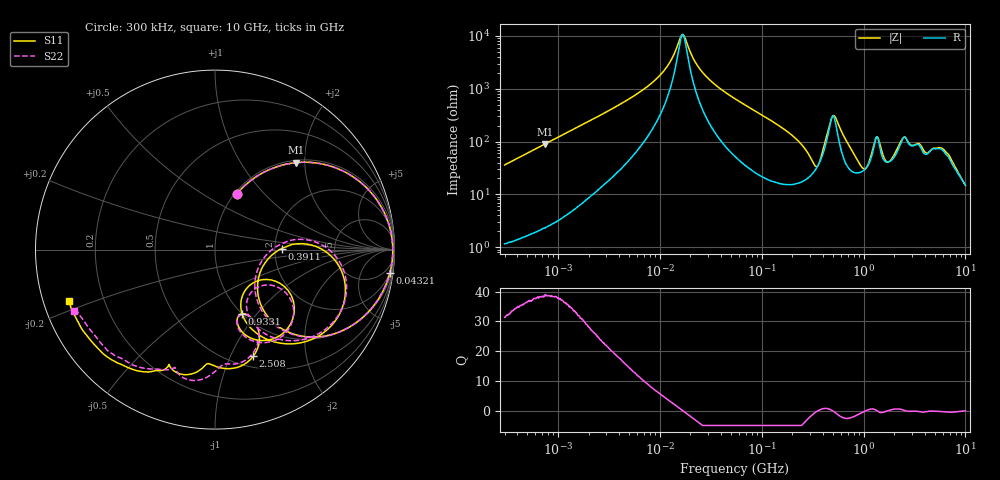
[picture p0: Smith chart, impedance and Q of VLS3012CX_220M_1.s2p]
! S-Parameter Data Generated by TDK Corporation
! Copyright(C) 2019 TDK Corporation.
! All Rights Reserved.
! TDK P/N: VLS3012CX-220M-1 (Inductor)
! Property: L=22uH at 1MHz
! Size(LxWxT): 3x3x1.2mm
! Model Type: s2p (Touchstone File Format Version 1.0)
! Frequency: DC=Yes Start=0.3MHz Stop=10000MHz 802points Log-sweep
! Model Generated on Sep. 23, 2019
! Port Assignments:
!  1 ---@@@--- 2
! Applicable Conditions:
!  Temperature = 25 degC
!  DC Bias Current = 0 A
!  Small Signal Operation
! Terms and conditions regarding TDK Simulation Models
! (1)This simulation model is being provided solely for informational purposes. Please refer to the specifications of the products in terms of detailed characteristics of such products.
! (2)In no event shall TDK Corporation of any of its subsidiaries be liable for any loss or damage arising, directly or indirectly,
!  From any information contained in this simulation model, including, but not limited to loss or damages arising from any inaccuracies, omissions or errors in connection with such information.
! (3)Any and all copyrights on this simulation model are owned by TDK Corporation.
!  Duplication or redistribution of this simulation model without prior written permission from TDK Corporation is prohibited.
! (4)This simulation model is subject to any modification or change without any prior notice.
! (5)Neither TDK Corporation nor any of its subsidiaries shall make any warranty, express or implied,
!  Including but not limited to the correctness, implied warranties of merchantability and fitness for a particular purpose with respect to this simulation models.
! (6)The use of this simulation model shall be deemed to have consented to the terms and conditions hereof.
# Hz S MA R 50
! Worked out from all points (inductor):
!   801 points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, 300 kHz to 10 GHz, reference 50 ohm
!   read as one part in series: L = 19.1 uH near 318.3 kHz
!   highest Q = 38.5 at 751 kHz (marker M1), where L = 19.1 uH
!   self-resonance near 16.72 MHz
!   S11 on the Smith chart (normalised r, x): 300 kHz: 1.02, +0.72; 43.21 MHz: 2, -15; 391.1 MHz: 2.18, +0.03; 933.1 MHz: 1.00, -0.84; 2.508 GHz: 0.62, -1.22; 10 GHz: 0.08, -0.17
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300000  0.3355 68.5  0.9313 -19.6  0.9315 -19.6  0.3353 68.6
750961  0.6606 47.1  0.7339 -41.4  0.734 -41.4  0.6605 47.2
1713600  0.8878 25.6  0.4324 -62.6  0.4324 -62.6  0.8877 25.6
9671944  0.9886 3.1  0.05928 -77.5  0.05929 -77.5  0.9887 3.1
1.694973e7  0.9907 -0.5  0.009324 5.9  0.009321 5.9  0.9908 -0.5
2.473055e7  0.9897 -3.0  0.0417 73.9  0.04169 73.9  0.9897 -3.0
4.320848e7  0.983 -7.6  0.1119 76.9  0.112 76.9  0.983 -7.6
5.477226e7  0.9766 -10.1  0.1507 75.3  0.1507 75.3  0.9765 -10.1
1.968335e8  0.7714 -38.8  0.5573 44.7  0.5573 44.7  0.7702 -39.0
3.126428e8  0.3852 -49.5  0.7586 11.0  0.7586 11.0  0.3761 -50.8
3.558009e8  0.2809 -23.2  0.7386 -4.7  0.7386 -4.7  0.2618 -23.0
3.910695e8  0.3715 0.9  0.6511 -17.7  0.6511 -17.7  0.3541 3.8
5.105874e8  0.7699 -19.7  0.2406 1.9  0.2406 1.9  0.7668 -17.1
6.656121e8  0.6838 -50.1  0.538 23.1  0.5381 23.1  0.6889 -47.1
9.330971e8  0.3873 -67.1  0.7311 -4.6  0.731 -4.6  0.4126 -63.0
1.117505e9  0.278 -44.7  0.7098 -23.6  0.7098 -23.6  0.3123 -44.5
1.323741e9  0.5455 -35.9  0.4384 -32.8  0.4383 -32.8  0.5641 -38.9
1.481453e9  0.5703 -62.7  0.5209 -13.4  0.5208 -13.4  0.5749 -64.3
1.767019e9  0.4099 -72.4  0.6391 -31.8  0.6389 -31.8  0.4136 -72.8
2.507534e9  0.6315 -70.3  0.3547 -54.6  0.3548 -54.6  0.6329 -73.1
6.010849e9  0.8006 -122.4  0.2542 -72.8  0.2542 -72.8  0.7756 -122.0
1e10  0.8633 -160.7  0.2135 -91.1  0.2134 -91.1  0.8591 -156.4
